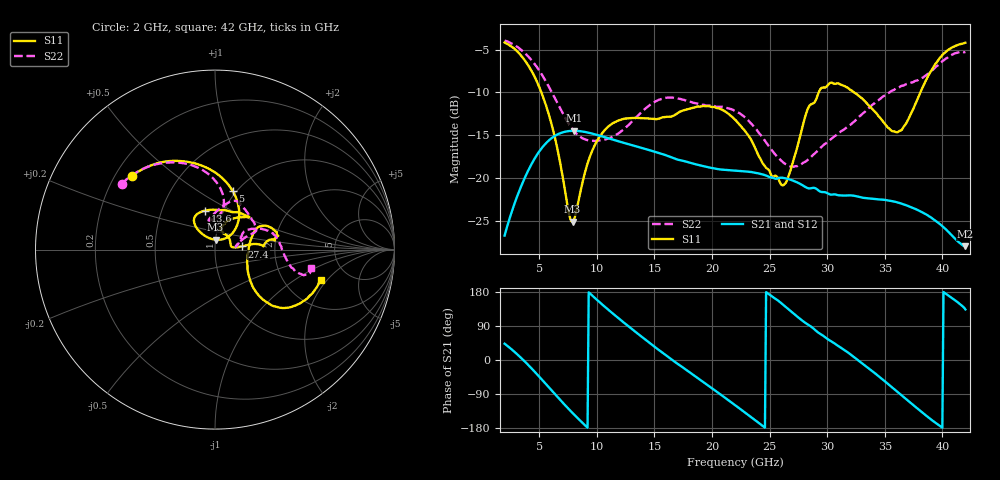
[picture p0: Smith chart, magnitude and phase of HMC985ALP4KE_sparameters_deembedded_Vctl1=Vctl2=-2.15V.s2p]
!s2p File: Measurements: S11, S21, S12, S22
# GHz S dB R 50.0
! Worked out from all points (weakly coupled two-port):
!   401 points, 2 GHz to 42 GHz, reference 50 ohm
!   highest |S21| = -14.48 dB at 8 GHz (marker M1); lowest = -28.0 dB at 42 GHz (marker M2)
!   lowest |S11| = -25.1 dB at 7.9 GHz (marker M3), VSWR 1.12, Z = 50 + j5.55 ohm
!   |S11| at or under -10 dB: 5.193 GHz to 29.27 GHz (24.08 GHz wide, 140 % of centre); 32.33 GHz to 38.09 GHz (5.763 GHz wide, 16.4 % of centre)
!   |S22| runs from -18.7 to -3.9 dB; largest |S21 - S12| = 0.0002
!   S11 on the Smith chart (normalised r, x): 2 GHz: 0.27, +0.36; 5 GHz: 0.96, +0.71; 13.6 GHz: 0.82, +0.37; 27.4 GHz: 1.35, +0.05; 42 GHz: 3.17, -1.76
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2  -4.16 138.5  -26.74 43.0  -26.73 43.0  -3.92 144.9
3.5  -5.81 107.3  -20.77 3.5  -20.77 3.5  -5.09 119.5
5  -9.35 73.2  -16.92 -43.8  -16.92 -43.8  -7.43 95.4
6.5  -16.07 44.9  -14.98 -94.6  -14.98 -94.6  -11.03 79.9
7.9  -25.13 86.6  -14.49 -139.9  -14.49 -139.9  -14.30 83.1
8  -24.94 94.7  -14.48 -143.0  -14.49 -143.0  -14.47 84.0
8.7  -20.88 125.2  -14.56 -164.1  -14.56 -164.1  -15.32 91.2
10.6  -14.55 127.9  -15.19 143.1  -15.20 143.1  -15.55 102.6
13.6  -12.99 104.2  -16.37 68.4  -16.38 68.4  -12.67 82.9
15.4  -13.06 81.4  -17.11 26.1  -17.11 26.1  -10.86 70.6
19  -11.65 44.6  -18.54 -52.7  -18.55 -52.8  -11.42 44.3
22  -13.17 54.4  -19.13 -119.0  -19.14 -119.0  -12.15 24.0
24.5  -18.45 75.4  -19.63 -176.2  -19.63 -176.2  -15.47 20.7
26.1  -20.87 16.7  -19.97 147.7  -19.98 147.7  -18.09 12.2
27.4  -16.45 6.7  -20.52 114.6  -20.52 114.5  -18.62 8.3
28.7  -11.33 3.9  -21.17 85.9  -21.18 85.9  -17.41 14.7
31.1  -9.04 16.5  -22.04 34.3  -22.04 34.3  -14.66 31.4
33.3  -11.07 27.3  -22.35 -14.8  -22.35 -14.8  -12.24 28.3
35.4  -14.24 7.7  -22.64 -66.2  -22.65 -66.2  -10.01 19.1
36.7  -13.90 -26.3  -23.12 -99.2  -23.12 -99.2  -9.15 11.1
39.4  -6.67 -43.1  -24.99 -165.5  -24.99 -165.5  -7.05 -13.5
42  -4.19 -16.1  -27.98 133.4  -27.98 133.4  -5.26 -10.6
